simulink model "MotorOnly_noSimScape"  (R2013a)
settings: Solver=ode23tb  StartTime=0  StopTime=2  FixedStep=1e-4  MaxStep=0.5e-3  RelTol=1e-3  AbsTol=1e-4
PreLoadFcn:
  | warning('off','sm:sli:setup:compile:LocalSolverNotSupported')
model workspace (MAT data in the model file):
  handle : class17 (value not decoded)
  handle : class17 (value not decoded)
undefined symbols (not defined in the file or in its folder): SimParamCB

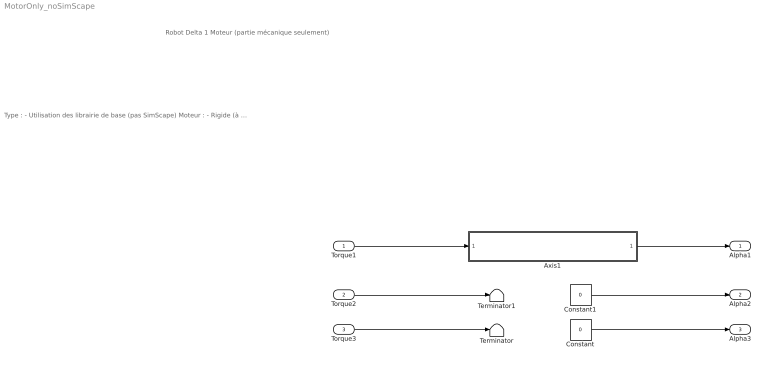
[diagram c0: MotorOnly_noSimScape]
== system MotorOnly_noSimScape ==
  note: Robot Delta 1 Moteur (partie mécanique seulement)
  note: Type : - Utilisation des librairie de base (pas SimScape) Moteur : - Rigide (à faire) - Rigide réducteur (à faire) - Flexible 1ddl (ok) Avec Volant d'inertie rigide
  Torque1 : Inport
  Torque2 : Inport  Port=2
  Torque3 : Inport  Port=3
  Axis1 : Subsystem
  Constant : Constant  Value=0
  Constant1 : Constant  Value=0
  Terminator : Terminator
  Terminator1 : Terminator
  Alpha1 : Outport
  Alpha2 : Outport  Port=2
  Alpha3 : Outport  Port=3
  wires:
  Axis1/1(Alpha) -> Alpha1/1
  Torque1/1 -> Axis1/1(Torque)
  Constant/1 -> Alpha3/1
  Torque3/1 -> Terminator/1
  Torque2/1 -> Terminator1/1
  Constant1/1 -> Alpha2/1

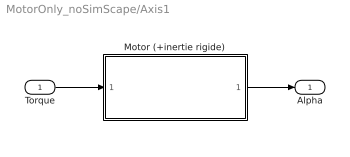
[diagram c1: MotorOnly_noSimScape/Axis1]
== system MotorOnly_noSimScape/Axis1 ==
  Torque : Inport
  Motor (+inertie rigide) : Subsystem  Variant=on
  Alpha : Outport
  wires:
  Motor (+inertie rigide)/1(Alpha) -> Alpha/1
  Torque/1 -> Motor (+inertie rigide)/1(Torque)

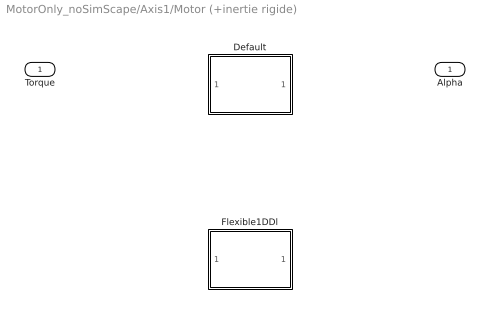
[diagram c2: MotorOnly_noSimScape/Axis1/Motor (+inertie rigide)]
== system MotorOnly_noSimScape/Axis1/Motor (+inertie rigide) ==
  Torque : Inport
  Default : Subsystem  VariantControl=motorVarDefault
  Flexible1DDl : Subsystem  InitFcn=SimParamCB = dummyCalbackText(RawParam);  VariantControl=motorVarFlex1
  Alpha : Outport

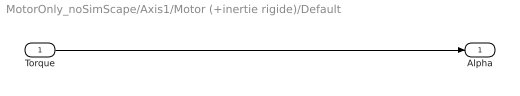
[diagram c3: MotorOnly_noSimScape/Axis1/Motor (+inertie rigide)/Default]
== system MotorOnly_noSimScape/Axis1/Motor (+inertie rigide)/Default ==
  Torque : Inport
  Alpha : Outport
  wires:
  Torque/1 -> Alpha/1

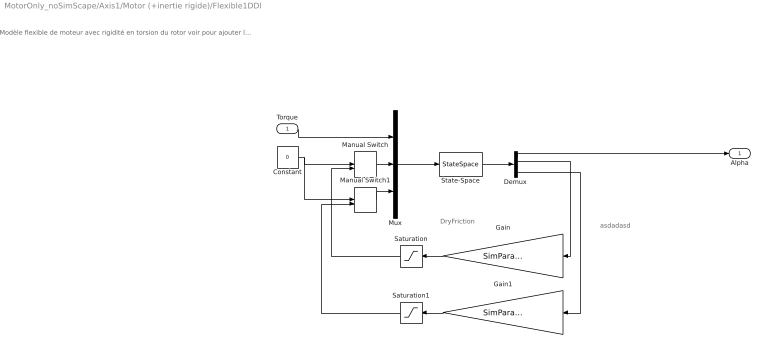
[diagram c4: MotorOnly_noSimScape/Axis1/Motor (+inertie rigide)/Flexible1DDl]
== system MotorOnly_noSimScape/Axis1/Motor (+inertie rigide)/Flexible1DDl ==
  note: Modèle flexible de moteur avec rigidité en torsion du rotor voir pour ajouter le frottement sec éventuellement
  note: asdadasd
  note: DryFriction
  Torque : Inport
  Constant : Constant  Value=0
  Demux : Demux
  Gain : Gain  Gain=SimParamCB.CdmotorSlope
  Gain1 : Gain  Gain=SimParamCB.CdmotorSlope
  Manual Switch : ManualSwitch  CurrentSetting=0
  Manual Switch1 : ManualSwitch  CurrentSetting=0
  Mux : Mux  Inputs=3
  Saturation : Saturate  UpperLimit=1  LowerLimit=-1
  Saturation1 : Saturate  UpperLimit=1  LowerLimit=-1
  State-Space : StateSpace  A=SimParamCB.Mec.A  B=SimParamCB.Mec.B  C=SimParamCB.Mec.C  D=SimParamCB.Mec.D
  Alpha : Outport
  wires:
  Gain/1 -> Saturation/1
  Saturation/1 -> Manual Switch/2
  Constant/1 -> Manual Switch/1, Manual Switch1/1
  State-Space/1 -> Demux/1
  Mux/1 -> State-Space/1
  Manual Switch/1 -> Mux/2
  Manual Switch1/1 -> Mux/3
  Demux/2 -> Gain/1
  Gain1/1 -> Saturation1/1
  Saturation1/1 -> Manual Switch1/2
  Demux/4 -> Gain1/1
  Demux/1 -> Alpha/1
  Torque/1 -> Mux/1
